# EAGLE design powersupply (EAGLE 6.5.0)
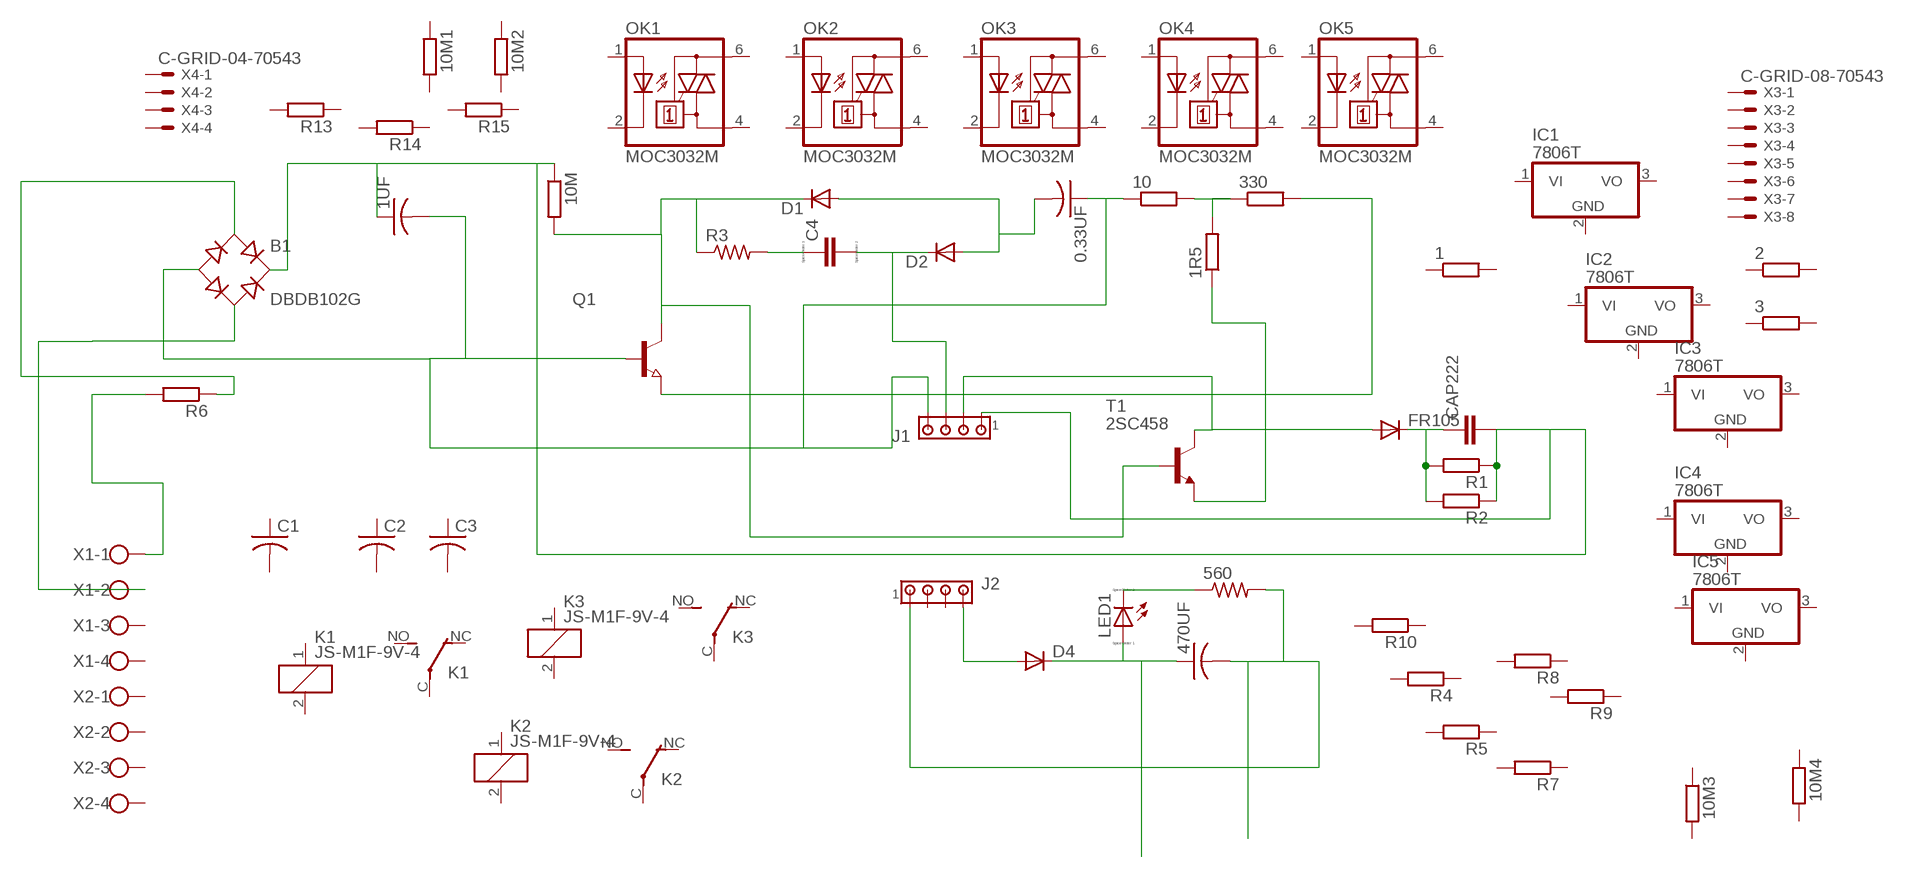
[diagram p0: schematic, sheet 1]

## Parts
0.33UF  C-US025-025X050  [C025-025X050]
1  R-EU_0207/7  [0207/7]
1R5  R-EU_0204/2V  [0204V]
1UF  C-US025-025X050  [C025-025X050]
2  R-EU_0207/7  [0207/7]
3  R-EU_0207/7  [0207/7]
10  R-EU_0207/5V  [0207/5V]
10M  R-EU_0207/7  [0207/7]
10M1  R-EU_0207/7  [0207/7]
10M2  R-EU_0207/7  [0207/7]
10M3  R-EU_0207/7  [0207/7]
10M4  R-EU_0207/7  [0207/7]
330  R-EU_0207/7  [0207/7]
470UF  C-US025-025X050  [C025-025X050]
560  R-US_0204/2V  [0204V]
B1  DBDB102G  [DB]
C1  C-US275-093X316  [C275-093X316]
C2  C-US275-093X316  [C275-093X316]
C3  C-US275-093X316  [C275-093X316]
C4  C  [C0805]
CAP222  C5/2.5  [C5B2.5]
D1  DIODE-D-2.5  [D-2.5]
D2  DIODE-D-2.5  [D-2.5]
D4  DIODE-D-5  [D-5]
FR105  DIODE-D-5  [D-5]
IC1  7806T  [TO220H]
IC2  7806T  [TO220H]
IC3  7806T  [TO220H]
IC4  7806T  [TO220H]
IC5  7806T  [TO220H]
J1  MTA04-100  [10X04MTA]
J2  MTA04-100  [10X04MTA]
K1  JS-M1F-9V-4  [JS-M]
K2  JS-M1F-9V-4  [JS-M]
K3  JS-M1F-9V-4  [JS-M]
LED1  LED_ELD260  [LED_LD260]
OK1  MOC3032M  [DIL06]
OK2  MOC3032M  [DIL06]
OK3  MOC3032M  [DIL06]
OK4  MOC3032M  [DIL06]
OK5  MOC3032M  [DIL06]
Q1  NPN-TRANSISTOR_SOT23  [SOT23]
R1  R-EU_0204/2V  [0204V]
R2  R-EU_0204/2V  [0204V]
R3  R-US_0204/2V  [0204V]
R4  R-EU_0204/2V  [0204V]
R5  R-EU_0204/2V  [0204V]
R6  R-EU_0204/2V  [0204V]
R7  R-EU_0204/2V  [0204V]
R8  R-EU_0204/2V  [0204V]
R9  R-EU_0204/2V  [0204V]
R10  R-EU_0204/2V  [0204V]
R13  R-EU_0204/2V  [0204V]
R14  R-EU_0204/2V  [0204V]
R15  R-EU_0204/2V  [0204V]
T1  2SC458  [TO92-ECB]
X1  W237-4  [W237-4]
X2  W237-4  [W237-4]
X3  C-GRID-08-70543  [70543-08]
X4  C-GRID-04-70543  [70543-04]

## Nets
N$1: B1.AC2 X1.2
N$2: B1.AC1 R6.1
N$4: 1UF.1 10M.1 B1.+ CAP222.2 J1.1 R1.1 R2.1
N$5: 1R5.1 T1.E
N$6: 10M.2 D1.C Q1.3(C) R3.1 T1.B
N$7: C4.1 R3.2
N$8: C4.2 D2.C J1.3
N$9: 0.33UF.2 D1.A D2.A
N$10: 0.33UF.1 1UF.2 10.1 B1.- J1.4 Q1.1(B)
N$11: 1R5.2 10.2 330.1
N$12: 330.2 Q1.2(E)
N$13: FR105.A J1.2 T1.C
N$14: CAP222.1 FR105.C R1.2 R2.2
N$16: R6.2 X1.1
N$17: D4.A J2.4
N$18: 470UF.1 D4.C LED1.A
N$19: 470UF.2 560.2 J2.1
N$20: 560.1 LED1.K(C)
Unconnected: 1.1 1.2 2.1 2.2 3.1 3.2 10M1.1 10M1.2 10M2.1 10M2.2 10M3.1 10M3.2 10M4.1 10M4.2 C1.1 C1.2 C2.1 C2.2 C3.1 C3.2 IC1.1(VI) IC1.2(GND) IC1.3(VO) IC2.1(VI) IC2.2(GND) IC2.3(VO) IC3.1(VI) IC3.2(GND) IC3.3(VO) IC4.1(VI) IC4.2(GND) IC4.3(VO) IC5.1(VI) IC5.2(GND) IC5.3(VO) J2.2 J2.3 K1.1 K1.2 K1.C(2:P) K1.NC(2:O) K1.NO(2:S) K2.1 K2.2 K2.C(2:P) K2.NC(2:O) K2.NO(2:S) K3.1 K3.2 K3.C(2:P) K3.NC(2:O) K3.NO(2:S) OK1.1(A) OK1.2(C) OK1.4(A1) OK1.6(A2) OK2.1(A) OK2.2(C) OK2.4(A1) OK2.6(A2) OK3.1(A) OK3.2(C) OK3.4(A1) OK3.6(A2) OK4.1(A) OK4.2(C) OK4.4(A1) OK4.6(A2) OK5.1(A) OK5.2(C) OK5.4(A1) OK5.6(A2) R4.1 R4.2 R5.1 R5.2 R7.1 R7.2 R8.1 R8.2 R9.1 R9.2 R10.1 R10.2 R13.1 R13.2 R14.1 R14.2 R15.1 R15.2 X1.3 X1.4 X2.1 X2.2 X2.3 X2.4 X3.1 X3.2 X3.3 X3.4 X3.5 X3.6 X3.7 X3.8 X4.1 X4.2 X4.3 X4.4

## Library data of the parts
0.33UF 1UF 470UF = rcl:C-US: CAPACITOR, American symbol
1 1R5 2 3 10 10M 10M1-10M4 330 R1 R2 R4-R10 R13-R15 = rcl:R-EU_: RESISTOR, European symbol
560 R3 = adafruit:R-US_: RESISTOR, American symbol
B1 = rectifier:DB?*G: Single Phase 1.0 AMP Glass Passivated Bridge Rectifier Taiwan Semiconductor Co.,Ltd. - TSC Source: http://www.taiwansemi.com/TSCbig5/ezcatfiles/cust/img/img/db101g.pdf http://www.ts.com.tw/db/pictures/modules/PDT/PDT060207001/DBLS201G.pdf
C1-C3 = adafruit:C-US: CAPACITOR, American symbol
C4 = eagle-ltspice:C: CAPACITOR, European symbol; SPICEMODEL: NONE; SPICEPREFIX: C
CAP222 = capacitor-wima:C: CAPACITOR
D1 D2 D4 FR105 = diode:DIODE-: DIODE
IC1-IC5 = adafruit:78*: Positive VOLTAGE REGULATOR Added bigger pads to the TO-92 package
J1 J2 = con-amp:MTA04-100: AMP connector
K1-K3 = relay:JS-M1*: Automotive Ultra-Miniature Power Relay NAiS Source: http://www.mew-europe.com/.. en_ds_61211_0000.pdf; OC_FARNELL: unknown; OC_NEWARK: unknown
LED1 = eagle-ltspice:LED_E: LED; SPICEMODEL: NONE; SPICEPREFIX: D; SPICETYPE: diode
OK1-OK5 = optocoupler:MOC30*: 6-Pin DIP Zero-Cross Optoisolators Triac Driver Output (250/400 Volt Peak) Source: The old path of data sheet not more available 2013-05-06.; MF: FAIRCHILD SEMICONDUCTOR; MPN: MOC3032-M; OC_FARNELL: 1203802; OC_NEWARK: 72K8897
Q1 = semicon-smd-ipc:NPN-TRANSISTOR_: NPN TRANSISTOR
T1 = transistor:2SC458: NPN Silicon Epitaxial Planar Transistor Source: SEMTECH ELECTRONICS LTD. ... 2SC458 1.pdf
X1 X2 = con-wago-500:W237-4: WAGO SCREW CLAMP; OC_FARNELL: unknown; OC_NEWARK: unknown
X3 = con-molex:C-GRID-08: CONNECTOR wire to board 2.54 mm (0.100") pitch header; OC_FARNELL: unknown; OC_NEWARK: unknown
X4 = con-molex:C-GRID-04: CONNECTOR wire to board 2.54 mm (0.100") pitch header; OC_FARNELL: unknown; OC_NEWARK: unknown

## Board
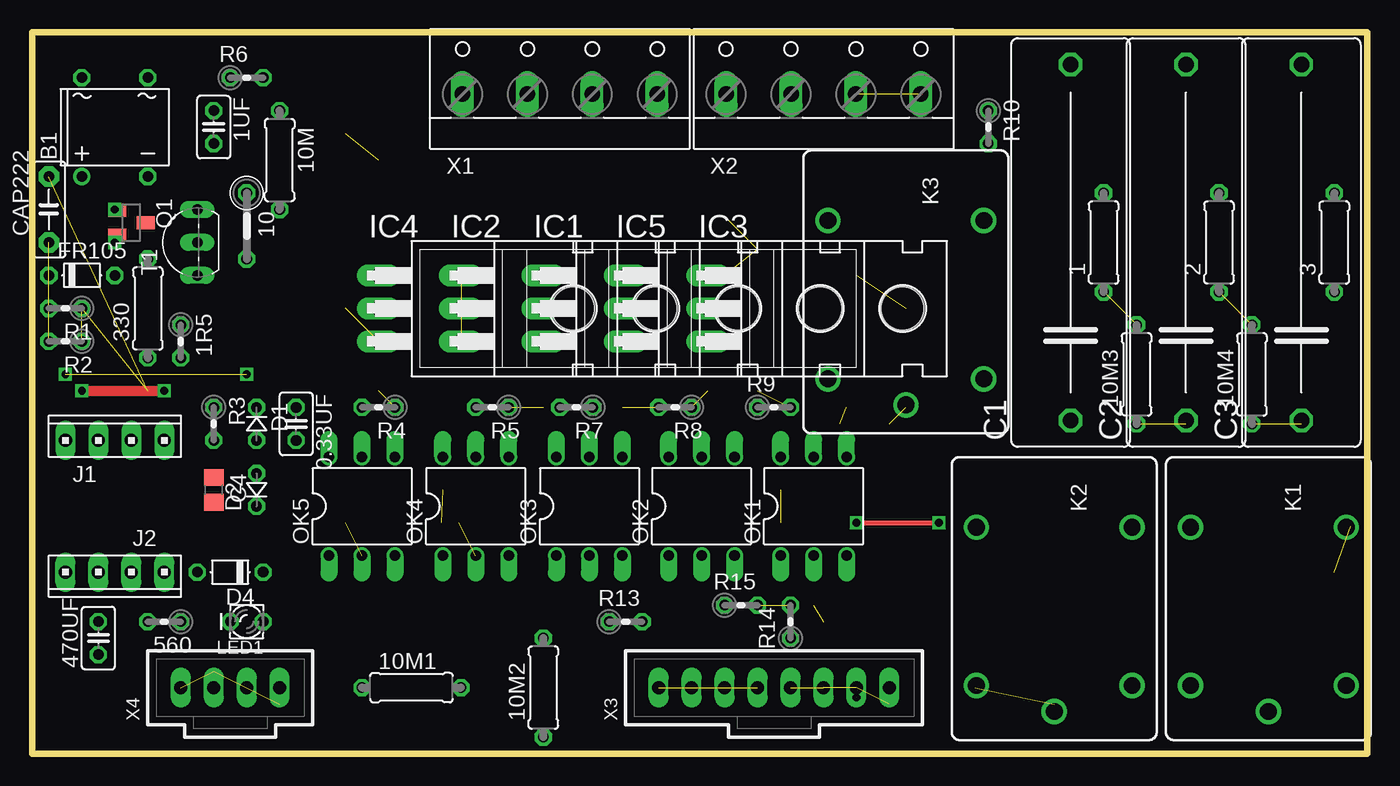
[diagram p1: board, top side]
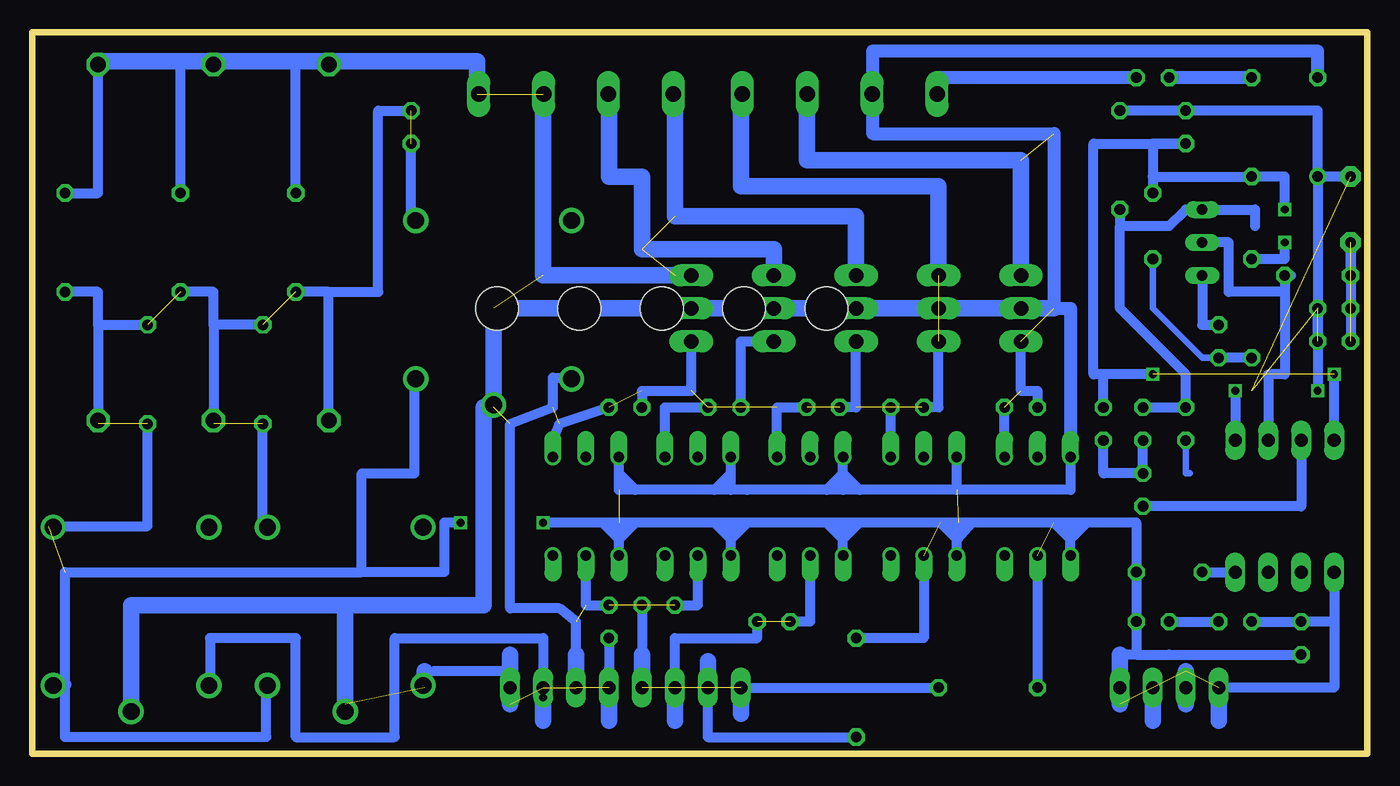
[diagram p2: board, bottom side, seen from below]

Size 102.85 x 55.55 mm. Coordinates in mm from the lower left corner, seen from the top.
Outline: 0,0 102.85,0 102.85,55.55 0,55.55 0,0
Copper layers (1*16): Top 0.035mm / dielectric 1.5mm / Bottom 0.035mm
Design rules "default": minimum track width 10mil, minimum drill 24mil, track to track 8mil, track to pad 8mil, pad to pad 8mil, via to via 8mil, smd to smd 8mil, copper to edge 40mil, drill to drill 8mil, minimum pad ring 10mil, minimum via ring 8mil, stop-mask expansion 4mil, vias tented up to drill 0mil, thermal gap 10mil

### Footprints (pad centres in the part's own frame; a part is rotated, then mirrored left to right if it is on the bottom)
C025-025X050 = drill 0.813 octagon: 1 -1.27,0; 2 1.27,0
0207/7 = drill 0.813 octagon: 1 -3.81,0; 2 3.81,0
0204V = drill 0.813 octagon: 1 -1.27,0; 2 1.27,0
0207/5V = drill 0.813 octagon: 1 -2.54,0; 2 2.54,0
DB = drill 0.813: + -2.54,-3.81 | drill 0.813 octagon: - 2.54,-3.81; AC1 2.54,3.81; AC2 -2.54,3.81
C275-093X316 = drill 1.194 octagon: 1 -13.716,0; 2 13.716,0
C0805 = smd 1.3 x 1.5: 1 -0.95,0; 2 0.95,0
C5B2.5 = drill 0.813 pad 1.6 octagon: 1 -2.54,0; 2 2.54,0
D-2.5 = drill 0.813 octagon: A 1.27,0; C -1.27,0
D-5 = drill 0.813 octagon: A 2.54,0; C -2.54,0
TO220H = drill 1.118 long: 1 -2.54,-10.16; 2 0,-10.16; 3 2.54,-10.16 | hole 3.302: 0,4.826
10X04MTA = drill 1.016 long: 1 3.81,0; 2 1.27,0; 3 -1.27,0; 4 -3.81,0
JS-M = drill 1.3: 1 6.7,6; 2 6.7,-6; C 8.7,0; NC -5.5,-6; NO -5.5,6
LED_LD260 = drill 0.813 octagon: A -1.27,0; K 1.27,0
DIL06 = drill 0.813 offset: 1 -2.54,-3.81; 2 0,-3.81; 3 2.54,-3.81; 4 2.54,3.81; 5 0,3.81; 6 -2.54,3.81
SOT23 = smd 1 x 1.4: 1 -0.95,-1.1; 2 0.95,-1.1; 3 0,1.1
TO92-ECB = drill 0.813 long: B 2.54,0; C 0,0; E -2.54,0
W237-4 = drill 1.194 long: 1 -7.5,-1.27; 2 -2.5,-1.27; 3 2.5,-1.27; 4 7.5,-1.27
70543-08 = drill 1.016 long: 1 -8.89,0; 2 -6.35,0; 3 -3.81,0; 4 -1.27,0; 5 1.27,0; 6 3.81,0; 7 6.35,0; 8 8.89,0
70543-04 = drill 1.016 long: 1 -3.81,0; 2 -1.27,0; 3 1.27,0; 4 3.81,0

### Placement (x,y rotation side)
0.33UF  20.32,25.4 270 top
1  82.55,39.37 90 top
1R5  11.43,31.75 270 top
1UF  13.97,48.26 270 top
2  91.44,39.37 90 top
3  100.33,39.37 90 top
10  16.51,40.64 270 top
10M  19.05,45.72 270 top
10M1  29.21,5.08 0 top
10M2  39.37,5.08 90 top
10M3  85.09,29.21 90 top
10M4  93.98,29.21 90 top
330  8.89,34.29 90 top
470UF  5.08,8.89 90 top
560  10.16,10.16 180 top
B1  6.35,48.26 0 top
C1  80.01,39.37 90 top
C2  88.9,39.37 90 top
C3  97.79,39.37 90 top
C4  13.97,20.32 270 top
CAP222  1.27,41.91 90 top
D1  17.27,25.4 270 top
D2  17.27,20.32 90 top
D4  15.24,13.97 180 top
FR105  3.81,36.83 0 top
IC1  49.53,34.29 270 top
IC2  43.18,34.29 270 top
IC3  62.23,34.29 270 top
IC4  36.83,34.29 270 top
IC5  55.88,34.29 270 top
J1  6.35,24.13 0 top
J2  6.35,13.97 180 top
K1  95.25,11.94 270 top
K2  78.74,11.94 270 top
K3  67.31,35.56 270 top
LED1  16.51,10.16 180 top
OK1  60.2,19.05 0 top
OK2  51.56,19.05 0 top
OK3  42.93,19.05 0 top
OK4  34.16,19.05 0 top
OK5  25.4,19.05 0 top
Q1  7.62,40.89 270 top
R1  2.54,34.29 180 top
R2  2.54,31.75 180 top
R3  13.97,25.4 270 top
R4  26.67,26.67 180 top
R5  35.43,26.67 180 top
R6  16.51,52.07 0 top
R7  41.91,26.67 180 top
R8  49.53,26.67 180 top
R9  57.15,26.67 0 top
R10  73.66,48.26 270 top
R13  45.72,10.16 0 top
R14  58.42,10.16 90 top
R15  54.61,11.43 0 top
T1  12.7,39.37 90 top
X1  40.64,52.07 0 top
X2  60.96,52.07 0 top
X3  57.15,5.08 0 top
X4  15.24,5.08 0 top

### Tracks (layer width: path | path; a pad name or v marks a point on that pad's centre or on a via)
N$1  (via drill 0.6)  (41 unrouted)
  Top 0.381: v63.5,17.78 v69.85,17.78
  Bottom 0.406: X1.2 38.1,50.8 38.1,54.1
  Bottom 0.762: 50.8,5.08 50.8,1.27 39.37,1.27 | 39.12,20.32 22.86,20.32 22.86,22.86 | 39.12,20.32 40.39,20.32 | 40.39,20.32 41.66,20.32 | 41.66,20.32 49.02,20.32 | 49.02,20.32 56.39,20.32 | 56.39,20.32 57.66,20.32 57.66,21.59 | 21.59,17.78 17.78,17.78 17.78,7.62 19.05,7.62 | 21.59,17.78 22.86,17.78 | 22.86,17.78 24.13,17.78 | 24.13,17.78 30.48,17.78 | 30.48,17.78 31.5,17.78 | 31.5,17.78 32.89,17.78 | 32.89,17.78 39.12,17.78 | 39.12,17.78 40.39,17.78 | 40.39,17.78 41.66,17.78 | 41.66,17.78 47.75,17.78 | 47.75,17.78 49.02,17.78 | 49.02,17.78 50.29,17.78 | 50.29,17.78 56.39,17.78 | 56.39,17.78 57.66,17.78 | 57.66,17.78 58.93,17.78 | 58.93,17.78 v63.5,17.78 | v69.85,17.78 71.12,17.78 71.12,13.97 77.47,13.97 | 84.84,5.08 84.84,1.27 100.33,1.27 100.33,5.33 100.33,13.97 77.47,13.97 | 77.47,13.97 77.47,21.59 73.41,21.59 73.41,29.21 | 48.26,5.08 33.02,5.08 | 53.34,5.08 53.34,8.89 46.99,8.89 46.99,10.16 | 53.34,11.43 51.56,11.43 51.56,15.24 | 58.42,8.89 58.42,5.08 | 60.96,7.62 60.96,10.16 62.23,11.18 66.04,11.18 66.04,25.4 62.74,26.67 62.74,28.96 60.96,28.96 | 31.62,20.32 31.62,22.86 | 40.39,20.32 40.39,21.59 | 40.39,21.59 40.39,22.86 | 49.02,20.32 49.02,22.86 | 57.66,21.59 57.66,22.86 | 57.66,13.97 57.66,16.51 | 57.66,16.51 57.66,17.78 | 49.02,13.97 49.02,16.51 | 49.02,16.51 49.02,17.78 | 40.39,13.97 40.39,16.51 | 40.39,16.51 40.39,17.78 | 31.62,13.97 31.62,16.51 | 31.62,16.51 32.89,17.78 | 22.86,13.97 22.86,16.51 | 22.86,16.51 22.86,17.78 | 27.94,22.86 27.94,26.67 | 26.67,31.75 26.67,27.94 25.4,27.94 25.4,26.67 | 36.7,22.86 36.7,26.67 | 33.02,31.75 33.02,26.67 34.29,26.67 | 45.47,22.86 45.47,26.67 43.18,26.67 | 54.1,22.86 54.1,26.67 50.8,26.67 | 62.74,22.86 62.74,24.13 62.23,25.4 58.42,26.67
  Bottom 0.762: 39.37,31.75 39.37,26.67 40.64,26.67 | 48.26,26.67 48.26,31.75 45.72,31.75 | 55.88,27.94 52.07,27.94 52.07,31.75 | 80.01,25.4 80.01,35.56 | 80.01,35.56 82.55,35.56 | 88.9,33.02 88.9,35.56 91.44,35.56 | 97.79,33.02 97.79,35.56 100.33,35.56 | 100.33,43.18 97.79,43.18 97.79,53.34 | 91.44,43.18 91.44,53.34 | 82.55,43.18 82.55,53.34 | 85.09,33.02 88.9,33.02 | 88.9,33.02 88.9,25.4 | 85.09,17.53 85.09,25.4 | 101.6,17.53 93.98,17.53 93.98,25.4 | 73.66,40.89 73.66,46.99 | 80.01,35.56 76.2,35.56 76.2,49.53 73.66,49.53 | 25.4,15.24 25.4,5.08 | 34.16,15.24 34.16,8.89 39.37,8.89 | 42.93,15.24 42.93,10.16 44.45,10.16 | 60.2,15.24 60.2,11.43 58.42,11.43 | 55.88,11.43 55.88,6.35 | 97.79,33.02 93.98,33.02 | 97.79,33.02 97.79,25.4 | 57.66,21.59 56.39,20.32 | 40.39,21.59 41.66,20.32 | 40.39,21.59 39.12,20.32 | 24.13,17.78 22.86,16.51 | 22.86,16.51 21.59,17.78 | 31.62,16.51 31.5,17.78 | 30.48,17.78 31.62,16.51 | 39.12,17.78 40.39,16.51 | 40.39,16.51 41.66,17.78 | 50.29,17.78 49.02,16.51 | 49.02,16.51 47.75,17.78 | 58.93,17.78 57.66,16.51 | 57.66,16.51 56.39,17.78
  Bottom 1.016: B1.AC2 3.81,54.1 38.1,54.1 38.1,47.75 24.13,47.75 24.13,34.29 22.86,34.29 22.86,22.86 | 101.6,5.33 100.33,5.33
  Bottom 1.27: 24.13,34.29 67.31,34.29 67.31,26.67 68.07,26.67 68.07,11.43 78.74,11.43 | 78.74,3.81 78.74,11.43 | 78.74,11.43 95.25,11.43 95.25,3.81 | 43.18,50.8 43.18,45.72 26.67,45.72 26.67,36.83 | 66.04,7.62 66.04,3.81 | 63.5,5.08 63.5,2.54 | 58.42,5.08 58.42,2.54 | 55.88,7.62 55.88,6.35 55.88,5.08 | 53.34,5.08 53.34,2.54 | 48.26,5.08 48.26,3.05 | 60.96,7.62 60.96,5.08 | 72.64,6.35 72.64,5.08 | 48.26,50.8 48.26,43.69 33.02,43.69 33.02,36.83 | 53.34,50.8 53.34,41.4 39.37,41.4 39.37,36.83 | 63.5,50.8 63.5,36.83 53.34,36.83 | 58.42,50.8 58.42,44.45 55.88,44.45 55.88,38.86 45.72,38.86 45.72,36.83 | 97.79,53.34 91.44,53.34 82.55,53.34 68.58,53.34 68.58,50.8 | 11.43,5.08 11.43,2.54 | 16.51,5.08 16.51,2.54 | 19.05,7.62 19.05,3.81 | 50.8,5.08 50.8,7.11 | 13.97,6.35 13.97,3.81
N$2
  Bottom 1.016: B1.AC1 R6.1
N$3
  Bottom 0.762: 47.75,20.32 50.29,20.32 49.02,21.59
N$4  (via drill 0.6)  (5 unrouted)
  Top 0.762: v3.81,27.94 v10.16,27.94
  Bottom 0.762: R1.1 v3.81,27.94 | v10.16,27.94 J1.1 | 10M.1 1UF.1 3.81,49.53 B1.+ | CAP222.2 B1.+ | B1.+ R1.1 | R2.1 R1.1
N$5
  Bottom 0.762: T1.E 12.7,33.02 1R5.1
N$6
  Bottom 0.762: 19.05,40.64 19.05,34.29 13.97,29.21 R3.1 D1.C | 10M.2 19.05,40.64 | 19.05,40.64 15.24,40.64 13.97,41.91 T1.B 8.64,41.91 8.64,40.64
N$7
  Bottom 0.508: R3.2 13.97,21.59 13.65,21.59
N$8  (via drill 0.6)  (2 unrouted)
  Bottom 0: 89.15,5.08 88.39,5.08
  Bottom 0.762: J1.3 5.08,19.05 D2.C | 66.04,6.35 71.88,6.35 | 89.15,5.08 89.15,8.89 82.55,8.89 82.55,1.27 74.93,1.27 74.93,8.89 63.5,8.89 63.5,6.86 v63.5,4.32
  other vias: 2.54,29.21 5.08,24.13 69.85,17.78
N$9
  Bottom 0.762: D1.A D2.A 20.32,21.59 0.33UF.2
N$10  (via drill 0.6)  (1 unrouted)
  Top 0.254: v6.35,41.91 Q1.1
  Bottom 0.762: 16.51,44.45 B1.- 6.35,44.45 v6.35,41.91 | J1.4 v2.54,29.21 | v16.51,29.21 20.32,29.21 | 0.33UF.1 20.32,29.21 | 20.32,29.21 21.08,29.21 21.08,46.99 1UF.2 16.51,46.99 16.51,44.45 | 16.51,44.45 10.1
N$11
  Bottom 0.508: 10.2 16.51,34.29 12.7,30.48 1R5.2
  Bottom 0.762: 330.1 1R5.2
N$12  (via drill 0.6)
  Top 0.254: v6.35,39.37 6.35,39.69 Q1.2
  Bottom 0.762: 330.2 6.35,38.1 v6.35,39.37
N$13
  Bottom 0.762: T1.C 10.67,39.37 10.67,35.56 6.35,35.56 FR105.A | 5.84,36.83 FR105.A | FR105.A 6.35,29.21 7.62,29.21 J1.2
N$14  (2 unrouted)
  Bottom 0.762: FR105.C CAP222.1 R1.2 R2.2
N$15
  Bottom 0.762: 55.88,27.94 55.88,26.67
N$16
  Bottom 0.406: X1.1 33.02,50.8
  Bottom 1.016: R6.2 33.02,52.07 33.02,50.8
N$17
  Bottom 0.762: D4.A J2.4
N$18
  Bottom 0.762: D4.C LED1.A 17.78,7.62 | 17.78,7.62 15.24,7.62 470UF.1 | 17.78,7.62 19.05,7.62 19.05,3.81
N$19
  Bottom 0.762: 560.2 470UF.2 2.54,10.16 | J2.1 2.54,10.16 | 2.54,10.16 2.54,5.08 11.43,5.08
N$20
  Bottom 0.762: LED1.K 560.1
